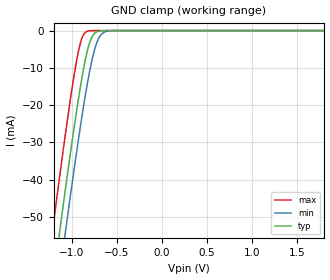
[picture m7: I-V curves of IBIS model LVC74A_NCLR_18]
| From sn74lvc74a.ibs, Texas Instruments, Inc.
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[Model]   LVC74A_NCLR_18
Model_type  Input
Vinl=0.5775
Vinh=1.2675
| variable   typ   min   max
C_comp   4.96pF   4.18pF   5.97pF
[Temperature Range]   40   100   -40
| Ambient temperature   25   85   -40
[Voltage range]   1.8   1.65   1.95
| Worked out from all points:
|   GND clamp passes 1 mA (typ) near -0.75 V on its own axis
[GND Clamp]
| LVC74A_NCLR_18
|   Voltage   I(typ)   I(min)   I(max)
-5.5V     -915.9mA   -925.7mA   -903.9mA
-1.215V   -69.33mA   -80.91mA   -54.47mA
-1.135V   -54.61mA   -66.2mA    -39.73mA
-1.075V   -43.82mA   -55.36mA   -29.01mA
-1.055V   -40.28mA   -51.8mA    -25.54mA
-955mV    -23.31mA   -34.48mA   -9.608mA
-885mV    -12.72mA   -23.13mA   -2.077mA
-825mV    -5.482mA   -14.34mA   -191.7uA
-780mV    -2.057mA   -8.704mA   -23.97uA
-715mV    -287.1uA   -2.975mA   -1.13uA
-650mV    -30.77uA   -620.5uA   -53.02nA
1.8V      3.327pA    7.106pA    3.026pA
